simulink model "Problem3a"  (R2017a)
settings: Solver=ode1  StartTime=0.0  StopTime=100  FixedStep=0.01  RelTol=1e-3
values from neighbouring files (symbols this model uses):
  Kp = 5    [Problem3.m]
  noise_var = 0.01    [Problem3.m]
  SP = 0    [Problem3.m]
  T = 10    [Problem3.m]
  tau = 2    [Problem3.m]
  tauf = 1    [Problem3.m]
libraries: simulink x1

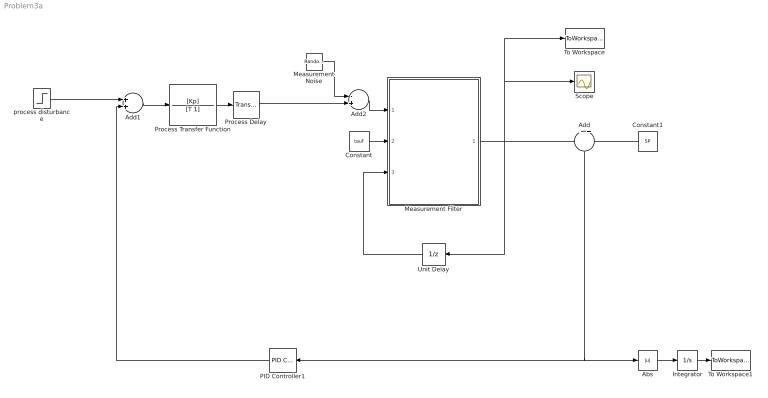
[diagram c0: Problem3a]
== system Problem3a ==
  Abs : Abs
  Add : Sum  Inputs=-+
  Add1 : Sum
  Add2 : Sum  Inputs=-+
  Constant : Constant  Value=tauf
  Constant1 : Constant  Value=SP
  Integrator : Integrator
  Measurement Noise : RandomNumber  Variance=noise_var  SampleTime=0.01
  Measurement Filter : MATLAB Function  TreatAsAtomicUnit=on
  PID Controller1 : simulink/Continuous/PID Controller  Controller=PID  TimeDomain=Continuous-time  SampleTime=-1  IntegratorMethod=Forward Euler  FilterMethod=Forward Euler  Form=Parallel  UseFilter=on  ControllerParametersSource=internal  P=0.34601608269574  I=0.042280920095562  D=0.256742591988959  N=0.378094165182863  InitialConditionSource=internal  InitialConditionForIntegrator=0  InitialConditionForFilter=0  ExternalReset=none  LimitOutput=off  UpperSaturationLimit=inf  LowerSaturationLimit=-inf  LinearizeAsGain=on  AntiWindupMode=none  Kb=1  TrackingMode=off  Kt=1  PParamMin=[]  PParamMax=[]  IParamMin=[]  IParamMax=[]  DParamMin=[]  DParamMax=[]  NParamMin=[]  NParamMax=[]  KbParamMin=[]  KbParamMax=[]  KtParamMin=[]  KtParamMax=[]  POutMin=[]  POutMax=[]  IOutMin=[]  IOutMax=[]  DOutMin=[]  DOutMax=[]  NOutMin=[]  NOutMax=[]  KbOutMin=[]  KbOutMax=[]  KtOutMin=[]  KtOutMax=[]  IntegratorOutMin=[]  IntegratorOutMax=[]  FilterOutMin=[]  FilterOutMax=[]  SumOutMin=[]  SumOutMax=[]  SumI1OutMin=[]  SumI1OutMax=[]  SumI2OutMin=[]  SumI2OutMax=[]  SumI3OutMin=[]  SumI3OutMax=[]  SumDOutMin=[]  SumDOutMax=[]  SaturationOutMin=[]  SaturationOutMax=[]  IntegratorContinuousStateAttributes=''  IntegratorStateMustResolveToSignalObject=off  IntegratorRTWStateStorageClass=Auto  FilterContinuousStateAttributes=''  FilterStateMustResolveToSignalObject=off  FilterRTWStateStorageClass=Auto  DifferentiatorICPrevScaledInput=0  DifferentiatorOutMin=[]  DifferentiatorOutMax=[]  InitialConditionSetting=State (most efficient)
  Process Delay : TransportDelay  DelayTime=tau
  Process Transfer Function : TransferFcn  Numerator=[Kp]  Denominator=[T 1]
  Scope : Scope
  To Workspace : ToWorkspace  VariableName=y  SaveFormat=Timeseries  SampleTime=-1
  To Workspace1 : ToWorkspace  VariableName=IAE  SampleTime=-1
  Unit Delay : UnitDelay  SampleTime=0.01
  process disturbance : Step  Time=10  SampleTime=0
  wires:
  Process Transfer Function/1 -> Process Delay/1
  Process Delay/1 -> Add2/2
  Constant/1 -> Measurement Filter/2(tau)
  Measurement Filter/1(ymeas) -> Add/1, To Workspace/1, Scope/1, Unit Delay/1
  Unit Delay/1 -> Measurement Filter/3(ut2)
  Constant1/1 -> Add/2
  PID Controller1/1 -> Add1/2
  process disturbance/1 -> Add1/1
  Add1/1 -> Process Transfer Function/1
  Add/1 -> PID Controller1/1, Abs/1
  Abs/1 -> Integrator/1
  Integrator/1 -> To Workspace1/1
  Measurement Noise/1 -> Add2/1
  Add2/1 -> Measurement Filter/1(ut1)

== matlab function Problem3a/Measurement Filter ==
function ymeas = fcn(ut1,tau, ut2)
alpha = 0.01/(tau+0.01);
ymeas = alpha*ut1+(1-alpha)*ut2;
